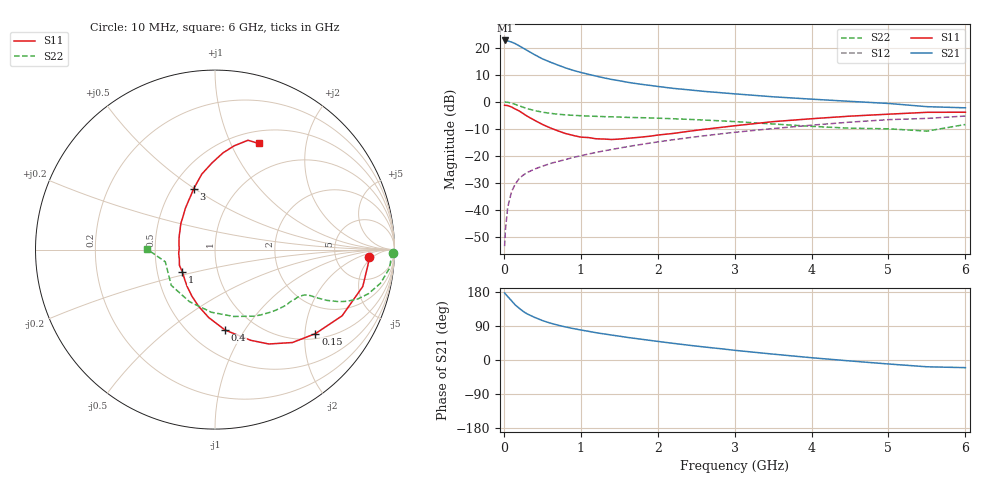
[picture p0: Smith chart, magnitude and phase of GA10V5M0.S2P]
! Infineon Technologies  Discrete & RF Semiconductors
! BF775
! Si NPN RF Bipolar Junction Transistor in SOT23
! VCE = 10 V  IC = 5 mA
! Common Emitter S-Parameters:  May  1996
# GHz  S  MA  R  50
!  f  S11  S21  S12  S22
! GHz  MAG  ANG  MAG  ANG  MAG  ANG  MAG  ANG
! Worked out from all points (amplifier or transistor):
!   36 points, 10 MHz to 6 GHz, reference 50 ohm
!   highest |S21| = 22.7 dB at 20 MHz (marker M1)
!   |S21| within 3 dB of that: start of sweep to 261.2 MHz
!   unconditionally stable (mu >= 1): 852.7 MHz to 2.918 GHz
!   at 250 MHz: K = 0.46, MSG = 23.6 dB, |S12| = -27.3 dB
!   at 1.4 GHz: K = 1.10, MAG = 11.1 dB, |S12| = -17.7 dB
!   at 6 GHz: K = 0.89, MSG = 1.5 dB, |S12| = -5.3 dB
!   S11 on the Smith chart (normalised r, x): 10 MHz: 12, -4; 150 MHz: 1.13, -2.27; 400 MHz: 0.73, -0.82; 1 GHz: 0.67, -0.18; 3 GHz: 0.64, +0.49; 6 GHz: 0.64, +1.28
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0.01  0.8614 -2.9  13.66 177.1  0.0021 83.5  0.9933 -1.1
0.02  0.857 -5.5  13.67 174.4  0.0041 86.8  0.9836 -2.4
0.05  0.8487 -14.0  13.4 167.6  0.011 83.4  0.9771 -6.2
0.1  0.7985 -27.5  12.77 156.3  0.0215 75.5  0.9408 -11.5
0.15  0.7297 -39.9  11.91 144.9  0.03 69.7  0.89 -16.0
0.2  0.6739 -50.2  10.86 136.5  0.0377 65.9  0.8416 -19.1
0.25  0.6054 -60.3  9.889 128.5  0.0434 62.9  0.7922 -21.3
0.3  0.5432 -68.5  8.986 122.0  0.0484 61.3  0.7481 -22.8
0.4  0.4521 -82.8  7.445 112.5  0.0565 58.5  0.6853 -24.4
0.5  0.3806 -95.2  6.258 104.2  0.0637 58.0  0.6411 -25.1
0.6  0.3286 -106.2  5.449 97.6  0.0712 58.2  0.6104 -25.5
0.8  0.2579 -126.9  4.25 87.3  0.0846 58.8  0.5711 -26.3
1  0.2206 -145.3  3.492 79.2  0.0996 59.6  0.5508 -27.6
1.1  0.2167 -156.2  3.223 75.7  0.1073 59.8  0.5427 -28.6
1.3  0.2035 -173.9  2.772 68.9  0.1228 60.0  0.5295 -30.3
1.6  0.2091 163.2  2.308 59.8  0.1462 59.8  0.5128 -34.0
2.2  0.2582 133.3  1.77 44.0  0.1972 57.4  0.4836 -43.2
3  0.3583 109.5  1.4 25.6  0.271 51.2  0.4284 -60.0
3.5  0.4272 99.9  1.234 15.5  0.3181 46.1  0.3867 -74.4
4.5  0.5405 85.3  1.016 -2.5  0.4186 34.5  0.3232 -116.0
5.5  0.6364 73.2  0.81 -17.9  0.4908 19.1  0.2849 -166.2
6  0.6394 67.6  0.771 -20.2  0.5431 14.8  0.3788 179.6
